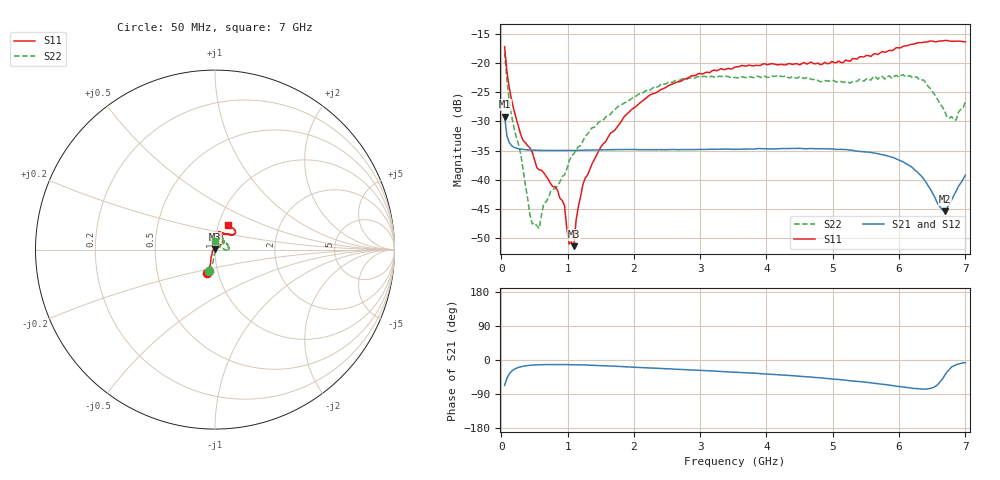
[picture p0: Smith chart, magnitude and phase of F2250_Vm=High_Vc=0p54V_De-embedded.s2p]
! Integrated Device Technology
! Corporate Headquarters
! 6024 Silver Creek Valley Road
! San Jose, CA 95138  USA
! Phone:  1-408-284-8200
! Toll Free:  1-800-223-1366
! Webpage:  http://www.idt.com/
! Timing and RF Division
! 515 Groton Road, Suite 102
! Westford, MA 01886-6024
! Device:  F2250
! Description: Voltage Variable RF Attenuator
! Frequency:  50.0 -  6000.00 MHz
! Package:  3x3 mm Thin QFN Plastic Package: 16 pin
! Ports:  2 RF, 3 DC
!  Pin  1  = GND
!  Pin  2  = NC
!  Pin  3  = RF1  = Port 1
!  Pin  4  = NC
!  Pin  5  = GND
!  Pin  6  = GND
!  Pin  7  = GND
!  Pin  8  = GND
!  Pin  9  = NC
!  Pin 10  = RF2  = Port 2
!  Pin 11  = NC
!  Pin 12  = GND
!  Pin 13  = GND
!  Pin 14  = VCNTRL
!  Pin 15  = VDD
!  Pin 16  = VMODE
! Vcntrl:  0.540 Volts
! Vmode:  +3.300 Volts
! Vdd:  +3.30  Volts
! Current:  1.272 mA
! Data:  The device was measured on a the F2250 evaluation board which has
!  individual transmission lines to the RF pins.  Data was collected
!  using a calibrated network analyzer.  The evaluation board was
!  de-embedded using a TRL calibration technique.
!  The reference plane is the edge of the package pin.
! Misc:  SN 10
!  Action Tracker AT0258
! Date Measured:  2014-11-26
! Date:  2015-10-15  MJV
! Note:
!  Integrated Device Technology supplies this data as a sample of measured
!  data at the package pin for this product.  Your particular data for this
!  product may vary.
!  Data was taken at 25 degrees C.
!  Integrated Device Technology reserves the right to change this data at anytime.
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# GHz S dB R 50
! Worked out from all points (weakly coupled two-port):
!   201 points, 50 MHz to 7 GHz, reference 50 ohm
!   highest |S21| = -29.16 dB at 50 MHz (marker M1); lowest = -45.5 dB at 6.687 GHz (marker M2)
!   lowest |S11| = -51.4 dB at 1.093 GHz (marker M3), VSWR 1.01, Z = 50 + j0.268 ohm
!   |S11| at or under -10 dB: start of sweep to end of sweep
!   |S22| runs from -48.4 to -18.2 dB; largest |S21 - S12| = 5.6e-05
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0.05  -17.17 -108.4  -29.16 -67.1  -29.16 -67.1  -18.15 -106.5
0.08475  -21.47 -107.3  -32.45 -48.0  -32.45 -48.0  -22.91 -98.8
0.189  -28.00 -119.8  -34.43 -25.1  -34.42 -25.1  -30.96 -97.6
0.328  -33.25 -133.8  -34.82 -16.5  -34.81 -16.5  -38.22 -80.6
0.467  -35.29 -145.9  -34.93 -13.5  -34.93 -13.5  -47.61 -60.0
0.57125  -38.33 -160.8  -34.97 -12.6  -34.97 -12.6  -48.41 -14.7
0.64075  -38.85 -162.3  -34.98 -12.2  -34.98 -12.2  -44.09 11.0
0.9535  -44.41 171.3  -35.01 -12.1  -35.01 -12.1  -39.20 34.4
1.023  -51.06 139.6  -35.00 -12.3  -35.00 -12.3  -36.84 31.8
1.0925  -51.43 87.3  -34.98 -12.5  -34.98 -12.5  -35.57 32.9
1.12725  -47.08 60.3  -34.97 -12.6  -34.97 -12.6  -34.92 29.7
1.2315  -40.79 39.9  -34.94 -13.0  -34.94 -13.0  -33.38 26.2
1.6485  -32.01 40.9  -34.87 -15.9  -34.87 -16.0  -28.76 32.6
1.96125  -27.99 40.6  -34.82 -18.7  -34.82 -18.7  -26.11 33.1
2.37825  -24.75 46.5  -34.85 -22.1  -34.85 -22.1  -23.96 38.7
3.525  -20.66 71.6  -34.79 -32.2  -34.80 -32.2  -22.46 64.2
4.7065  -20.07 71.9  -34.67 -45.7  -34.67 -45.7  -22.80 65.0
5.85325  -17.80 40.5  -36.03 -66.3  -36.03 -66.5  -22.18 15.1
6.3745  -16.40 40.9  -39.91 -76.8  -39.91 -77.0  -22.92 -1.4
6.68725  -16.12 47.8  -45.47 -40.6  -45.45 -40.3  -28.23 20.7
6.861  -16.22 54.5  -41.99 -12.4  -41.95 -12.6  -29.75 59.1
7  -16.33 62.4  -39.23 -7.1  -39.20 -7.3  -26.48 91.0
